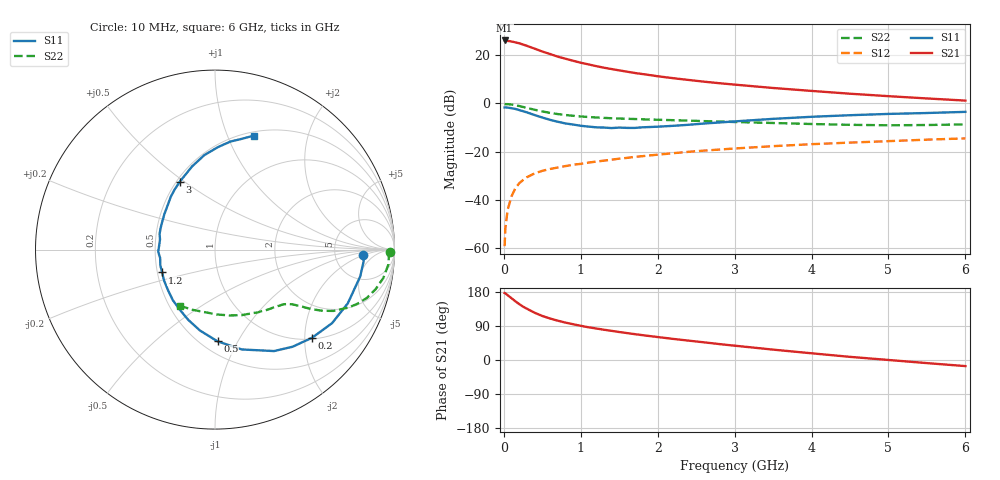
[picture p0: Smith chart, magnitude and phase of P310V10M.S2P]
! SIEMENS Small Signal Semiconductors
! BFP181
! Si NPN RF Bipolar Junction Transistor in SOT143
! VCE = 10 V  IC = 10 mA
! Common Emitter S-Parameters:  March  1996
# GHz  S  MA  R  50
!  f  S11  S21  S12  S22
! GHz  MAG  ANG  MAG  ANG  MAG  ANG  MAG  ANG
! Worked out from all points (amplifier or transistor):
!   36 points, 10 MHz to 6 GHz, reference 50 ohm
!   highest |S21| = 26.1 dB at 10 MHz (marker M1)
!   |S21| within 3 dB of that: start of sweep to 365.9 MHz
!   unconditionally stable (mu >= 1): 1.385 GHz to end of sweep
!   at 250 MHz: K = 0.31, MSG = 28.1 dB, |S12| = -31.7 dB
!   at 1.4 GHz: K = 1.00, MAG = 18.4 dB, |S12| = -23.3 dB
!   at 6 GHz: K = 1.05, MAG = 6.5 dB, |S12| = -14.5 dB
!   S11 on the Smith chart (normalised r, x): 10 MHz: 10, -2; 200 MHz: 1.03, -2.18; 500 MHz: 0.60, -0.83; 1.2 GHz: 0.53, -0.15; 3 GHz: 0.52, +0.48; 6 GHz: 0.54, +1.25
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0.01  0.8259 -2.1  20.29 176.8  0.0011 61.4  0.9752 -0.7
0.02  0.831 -4.4  20.07 176.0  0.0026 87.3  0.9697 -1.8
0.05  0.8227 -10.5  19.87 171.0  0.0063 85.0  0.9697 -4.9
0.1  0.7983 -22.0  19.3 163.0  0.0119 75.5  0.951 -9.6
0.15  0.7705 -32.1  18.52 154.9  0.0175 70.9  0.9213 -13.9
0.2  0.7308 -42.2  17.73 147.6  0.0222 68.7  0.8873 -17.7
0.25  0.6926 -51.4  16.67 140.8  0.0259 64.6  0.8477 -20.9
0.3  0.6541 -59.8  15.69 135.3  0.0296 61.2  0.8103 -23.5
0.4  0.5763 -74.9  13.72 124.7  0.0355 57.1  0.7425 -27.4
0.5  0.5115 -88.4  11.96 116.2  0.0401 53.1  0.685 -29.8
0.6  0.4587 -100.5  10.62 109.5  0.0438 52.0  0.6385 -31.4
0.7  0.4187 -110.9  9.375 103.8  0.0471 50.2  0.6039 -32.5
0.8  0.3862 -121.1  8.487 98.7  0.0503 49.4  0.5771 -33.3
1.1  0.3322 -148.7  6.478 86.4  0.0595 48.1  0.5243 -35.5
1.2  0.3206 -156.6  5.959 83.2  0.0624 47.6  0.5134 -36.3
1.7  0.3115 169.6  4.3 68.3  0.0782 46.4  0.4767 -41.0
2.2  0.3442 145.2  3.349 55.7  0.0932 44.0  0.4508 -47.0
3  0.4252 117.7  2.463 37.8  0.1166 38.6  0.4128 -58.9
3.5  0.4802 105.5  2.098 27.4  0.1304 34.8  0.3942 -67.9
4.5  0.5715 88.3  1.596 8.3  0.1546 26.7  0.3614 -88.6
5.5  0.6349 76.4  1.273 -8.2  0.178 19.8  0.358 -110.5
6  0.6707 71.2  1.149 -16.1  0.189 15.8  0.3686 -121.9
